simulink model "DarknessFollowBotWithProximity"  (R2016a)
settings: Solver=FixedStepAuto  StartTime=0.0  StopTime=10.0  RelTol=1e-3
libraries: miniQ x3

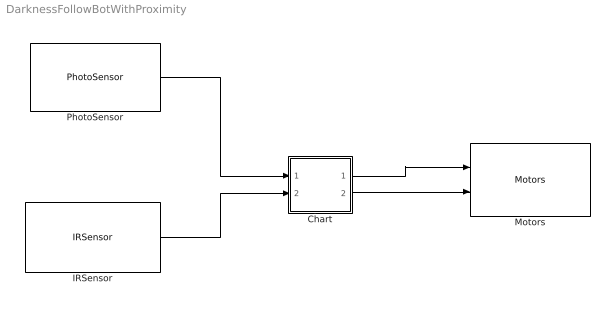
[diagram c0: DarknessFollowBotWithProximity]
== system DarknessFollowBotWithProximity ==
  Chart : Stateflow chart  TreatAsAtomicUnit=on
  IRSensor : miniQ/IRSensor  sampleTime_dd=0.01  debug_dd=off
  Motors : miniQ/Motors  flipLeft=off  flipRight=off
  PhotoSensor : miniQ/PhotoSensor  sampleTime_dd=0.01  debug_dd=off
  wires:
  PhotoSensor/1 -> Chart/1(lite)
  Chart/1(l) -> Motors/1
  Chart/2(r) -> Motors/2
  IRSensor/1 -> Chart/2(prox)

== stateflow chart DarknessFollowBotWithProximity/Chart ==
  state Stop
    entry: l=0
    r=0
  state Forward
    entry: l= 255
    r=255
  state Right
    entry: l=-200
    r=200
  state Left
    entry: l=200
    r=-200
  (default) -> Stop
  Left -> Stop : [prox<2]
  Forward -> Stop : [prox<2]
  Stop -> Forward : [prox>30]
  Right -> Stop : [prox<2]
  Right -> Forward : [lite<800]
  Left -> Forward : [lite>40]
  Forward -> Left : [lite<40]
  Forward -> Right : [lite>400]
  data: l output; r output; lite input; prox input
